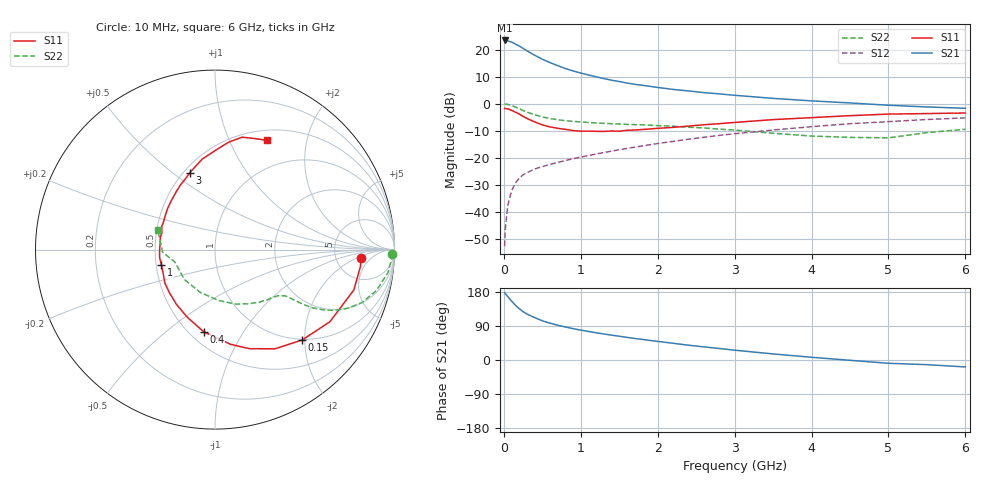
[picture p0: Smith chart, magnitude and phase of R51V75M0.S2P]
! SIEMENS Small Signal Semiconductors
! BFR183
! Si NPN RF Bipolar Junction Transistor in SOT23
! VCE = 1.75 V  IC = 5 mA
! Common Emitter S-Parameters:  May  1996
# GHz  S  MA  R  50
!  f  S11  S21  S12  S22
! GHz  MAG  ANG  MAG  ANG  MAG  ANG  MAG  ANG
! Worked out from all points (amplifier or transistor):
!   36 points, 10 MHz to 6 GHz, reference 50 ohm
!   highest |S21| = 23.5 dB at 10 MHz (marker M1)
!   |S21| within 3 dB of that: start of sweep to 254.6 MHz
!   unconditionally stable (mu >= 1): 1.006 GHz to 2.684 GHz
!   at 250 MHz: K = 0.43, MSG = 23.4 dB, |S12| = -26.3 dB
!   at 1.4 GHz: K = 1.07, MAG = 11.6 dB, |S12| = -17.6 dB
!   at 6 GHz: K = 0.90, MSG = 1.8 dB, |S12| = -5.2 dB
!   S11 on the Smith chart (normalised r, x): 10 MHz: 9.16, -2.58; 150 MHz: 0.99, -1.95; 400 MHz: 0.59, -0.68; 1 GHz: 0.53, -0.10; 3 GHz: 0.54, +0.58; 6 GHz: 0.62, +1.39
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0.01  0.8164 -3.3  14.89 177.6  0.0023 85.8  0.9891 -1.5
0.02  0.8156 -6.7  14.76 174.8  0.005 83.6  0.9845 -3.1
0.05  0.8057 -16.2  14.56 167.4  0.0128 80.6  0.9727 -7.5
0.1  0.756 -32.1  13.98 155.6  0.0243 74.7  0.9282 -14.2
0.15  0.6999 -46.0  12.76 144.5  0.0339 67.9  0.8706 -19.8
0.2  0.6461 -58.8  11.74 135.6  0.0418 63.5  0.8111 -23.7
0.25  0.5845 -70.8  10.65 127.6  0.0482 59.5  0.7503 -26.8
0.3  0.5353 -80.6  9.59 121.3  0.053 58.1  0.7009 -28.8
0.4  0.4623 -97.8  7.941 111.9  0.0616 55.1  0.6269 -31.0
0.5  0.4059 -112.7  6.682 103.5  0.0686 54.6  0.571 -31.9
0.6  0.3734 -125.0  5.79 97.2  0.0751 54.5  0.5326 -32.4
0.8  0.3357 -146.4  4.495 87.1  0.0886 55.3  0.4852 -33.0
1  0.3105 -164.0  3.704 78.8  0.1026 56.5  0.4605 -33.9
1.1  0.3117 -172.1  3.416 75.4  0.11 57.0  0.4499 -34.9
1.3  0.3074 173.9  2.927 68.7  0.125 57.8  0.4332 -36.5
1.6  0.3233 156.6  2.422 59.7  0.1489 57.8  0.4145 -40.1
2.2  0.3657 131.6  1.844 44.1  0.201 55.7  0.3843 -49.8
3  0.4509 108.2  1.436 25.9  0.2789 49.2  0.3262 -68.8
3.5  0.509 98.1  1.259 16.0  0.3264 43.7  0.2841 -86.0
4.5  0.6023 82.9  1.036 -0.8  0.4278 31.4  0.2383 -135.6
5.5  0.6581 70.0  0.873 -12.3  0.5109 18.9  0.2919 -177.1
6  0.6743 64.5  0.825 -18.3  0.5491 10.7  0.337 161.0
